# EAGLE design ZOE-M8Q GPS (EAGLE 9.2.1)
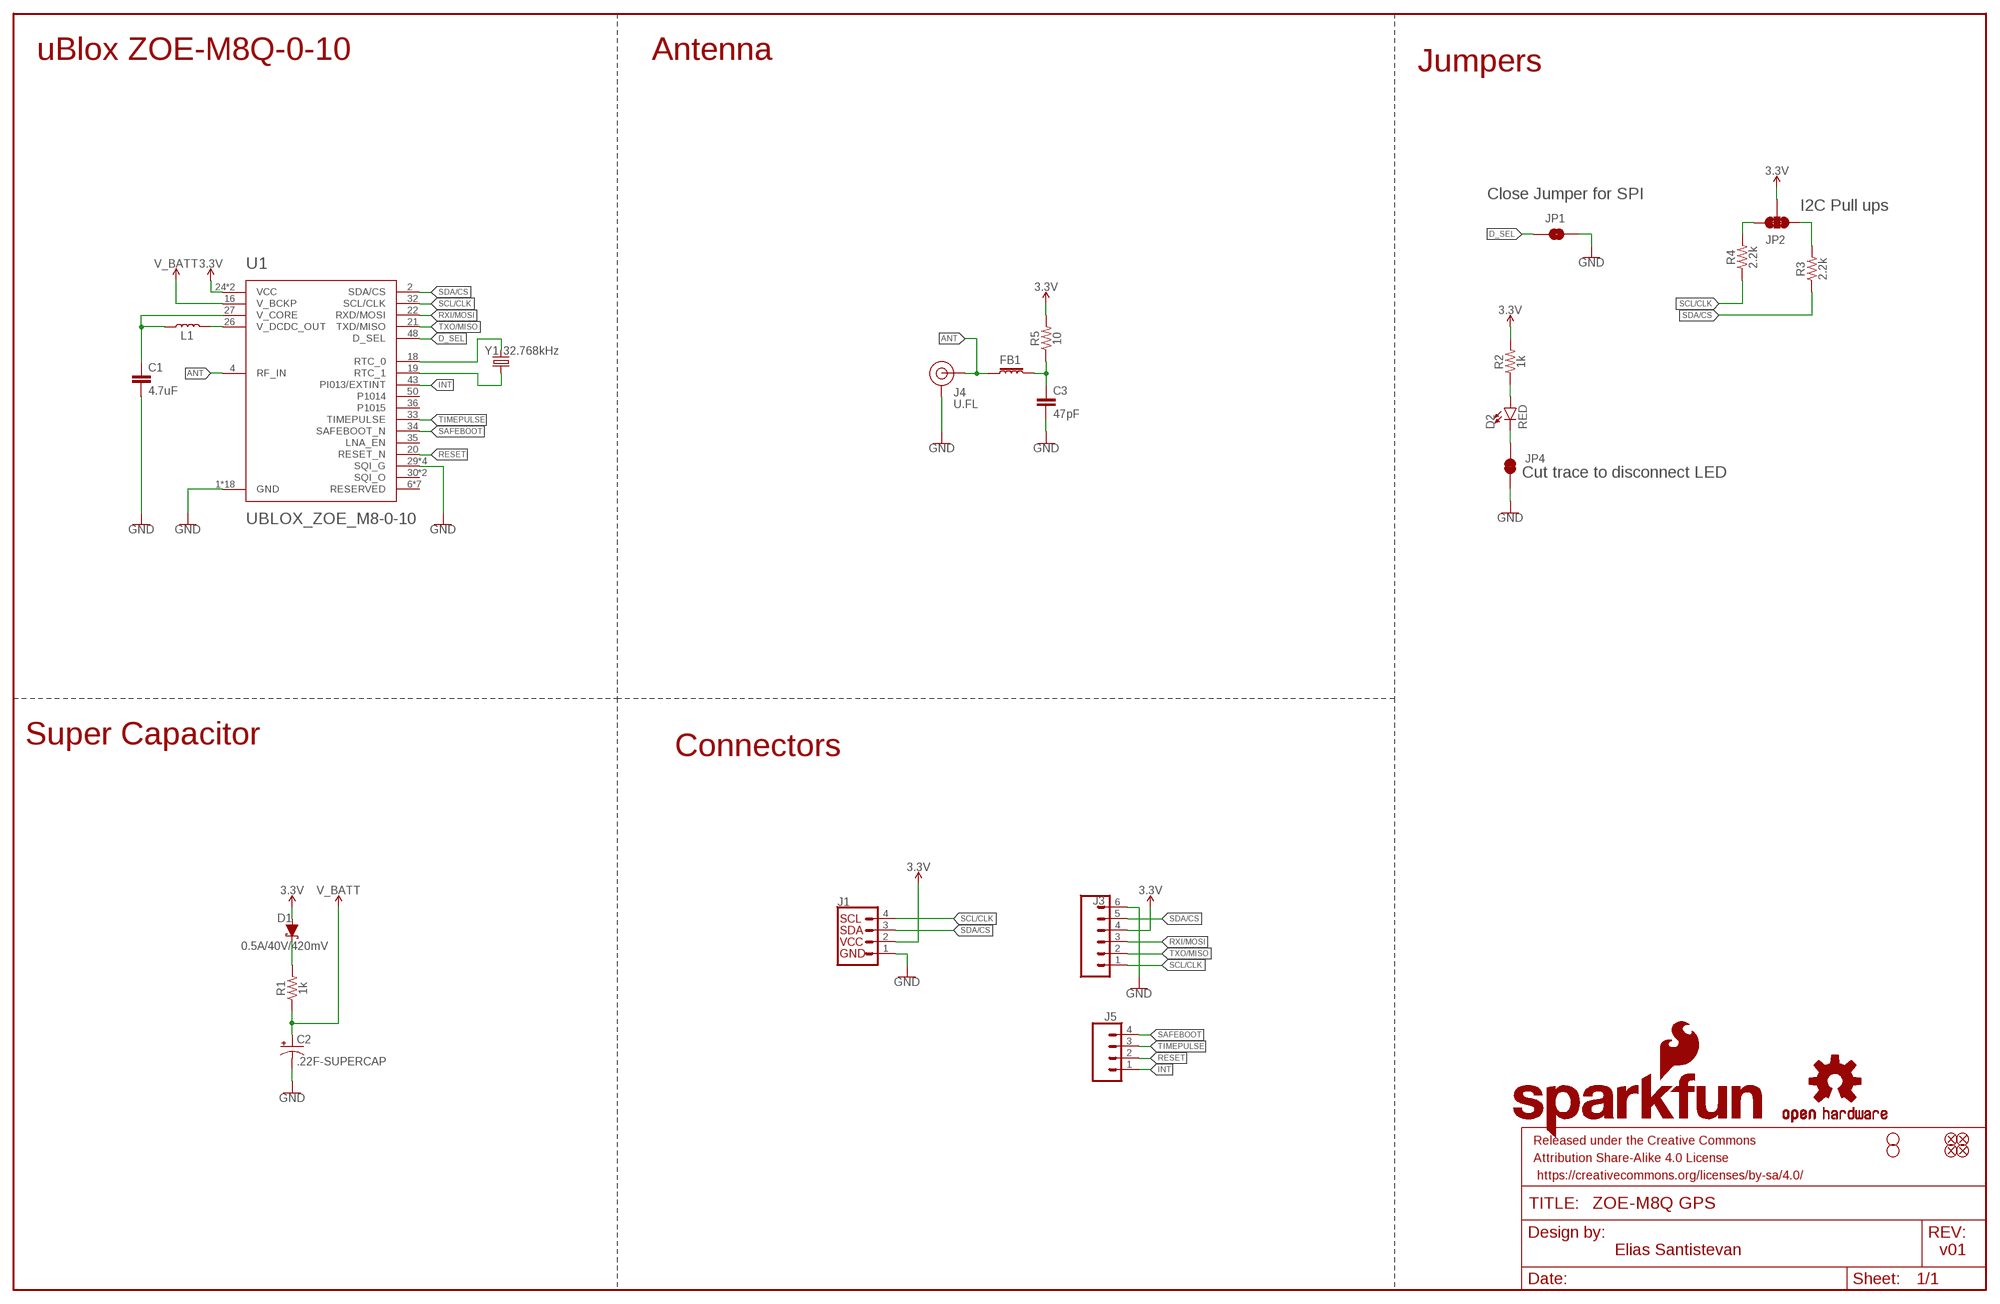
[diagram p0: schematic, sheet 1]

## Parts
C1  4.7uF  4.7UF-0603-6.3V-(10%)  [0603]
C2  .22F-SUPERCAP  [DSK-RADIAL-4.8MM]
C3  47pF  47PF-0603-50V-5%  [0603]
D1  0.5A/40V/420mV  DIODE-SCHOTTKY-PMEG4005EJ  [SOD-323]
D2  RED  LED-RED0603  [LED-0603]
FB1  FERRITE_BEAD-120_OHM-0402  [0402]
FD1  FIDUCIALUFIDUCIAL  [FIDUCIAL-MICRO]
FD2  FIDUCIALUFIDUCIAL  [FIDUCIAL-MICRO]
FD3  FIDUCIALUFIDUCIAL  [FIDUCIAL-MICRO]
FD4  FIDUCIALUFIDUCIAL  [FIDUCIAL-MICRO]
FRAME1  FRAME-LEDGER  [CREATIVE_COMMONS]
H2  STAND-OFFTIGHT  [STAND-OFF-TIGHT]
H3  STAND-OFFTIGHT  [STAND-OFF-TIGHT]
J1  QWIIC_CONNECTORJS-1MM  [JST04_1MM_RA]
J3  CONN_06NO_SILK_NO_POP  [1X06_NO_SILK]
J4  U.FL  U.FL2PIN  [U.FL]
J5  CONN_041X04_NO_SILK  [1X04_NO_SILK]
JP1  JUMPER-SMT_2_NO_SILK  [SMT-JUMPER_2_NO_SILK]
JP2  JUMPER-SMT_3_2-NC_TRACE_SILK  [SMT-JUMPER_3_2-NC_TRACE_SILK]
JP4  JUMPER-SMT_2_NC_TRACE_SILK  [SMT-JUMPER_2_NC_TRACE_SILK]
L1  2.2UH_SHIELDED_INDUCTOR  [0806_NDUC]
LOGO1  SFE_LOGO_NAME_FLAME.1_INCH  [SFE_LOGO_NAME_FLAME_.1]
LOGO2  OSHW-LOGOS  [OSHW-LOGO-S]
LOGO3  SFE_LOGO_FLAME.1_INCH  [SFE_LOGO_FLAME_.1]
R1  1k  1KOHM-0603-1/10W-1%  [0603]
R2  1k  1KOHM-0603-1/10W-1%  [0603]
R3  2.2k  2.2KOHM-0603-1/10W-1%  [0603]
R4  2.2k  2.2KOHM-0603-1/10W-1%  [0603]
R5  10  10OHM-0603-1/10W-1%  [0603]
U1  UBLOX_ZOE_M8-0-10  [UBLOX_ZOE_M8-0-10]
Y1  32.768kHz  CRYSTAL-32.768KHZSMD-3.2X1.5  [CRYSTAL-SMD-3.2X1.5MM]

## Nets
3.3V: D1.A J1.2 J3.4 JP2.2 R2.2 R5.2 U1.24(VCC) U1.25(VCC)
ANT: FB1.1 J4.FEED(SIGNAL) U1.4(RF_IN)
D_SEL: JP1.1 U1.48(D_SEL)
GND: C1.2 C2.- C3.2 J1.1 J3.6 J4.1(GND) J4.2(GND) JP1.2 JP4.1 U1.1(GND) U1.3(GND) U1.5(GND) U1.7(GND) U1.8(GND) U1.9(GND) U1.10(GND) U1.11(GND) U1.12(GND) U1.17(GND) U1.23(GND) U1.29(SQI_G) U1.31(SQI_G) U1.37(GND) U1.38(GND) U1.39(GND) U1.40(GND) U1.41(GND) U1.44(GND) U1.46(SQI_G) U1.47(SQI_G) U1.49(GND)
INT: J5.1 U1.43(PI013/EXTINT)
N$1: JP2.1 R3.2
N$2: D1.C R1.2
N$3: JP2.3 R4.2
N$4: D2.A R2.1
N$6: C1.1 L1.P$1 U1.27(V_CORE)
N$7: L1.P$2 U1.26(V_DCDC_OUT)
N$8: D2.C JP4.2
N$9: C3.1 FB1.2 R5.1
N$13: U1.18(RTC_0) Y1.P$2
N$15: U1.19(RTC_1) Y1.P$1
RESET: J5.2 U1.20(RESET_N)
RXI/MOSI: J3.3 U1.22(RXD/MOSI)
SAFEBOOT: J5.4 U1.34(SAFEBOOT_N)
SCL/CLK: J1.4 J3.1 R4.1 U1.32(SCL/CLK)
SDA/CS: J1.3 J3.5 R3.1 U1.2(SDA/CS)
TIMEPULSE: J5.3 U1.33(TIMEPULSE)
TXO/MISO: J3.2 U1.21(TXD/MISO)
V_BATT: C2.+ R1.1 U1.16(V_BCKP)
Unconnected: U1.6(RESERVED) U1.13(RESERVED) U1.14(RESERVED) U1.15(RESERVED) U1.28(RESERVED) U1.30(SQI_O) U1.35(LNA_EN) U1.36(P1015) U1.42(RESERVED) U1.45(SQI_O) U1.50(P1014) U1.51(RESERVED)

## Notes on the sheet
- uBlox ZOE-M8Q-0-10 | Antenna
- Jumpers
- Close Jumper for SPI
- I2C Pull ups
- Cut trace to disconnect LED
- Super Capacitor
- Connectors
- Elias Santistevan | v01

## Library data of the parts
C1 = SparkFun-Capacitors:4.7UF: 4.7µF ceramic capacitors; PROD_ID: CAP-08280
C2 = SparkFun-Capacitors:.22F-SUPERCAP: ELNA DSK-621 - 220mF Electric Double Layer Capacitor (EDLC/SuperCapacitor); PROD_ID: CAP-13907
C3 = SparkFun-Capacitors:47PF: 47pF ceramic capacitors; PROD_ID: CAP-08913
D1 = SparkFun-DiscreteSemi:DIODE-SCHOTTKY: Schottky diode; PROD_ID: DIO-10955
D2 = SparkFun-LED:LED-RED: Red SMD LED; PROD_ID: DIO-00819
FB1 = SparkFun-Coils:FERRITE_BEAD-120_OHM: Ferrite Bead (blocks, cores, rings, chokes, etc.); MFG_PART: BLM15HB121SN1D; PROD_ID: NDUC-14206
FD1-FD4 = SparkFun-Aesthetics:FIDUCIAL: Fiducial Alignment Points
FRAME1 = SparkFun-Aesthetics:FRAME-LEDGER: Schematic Frame - Ledger
H2 H3 = SparkFun-Hardware:STAND-OFF: Stand Off
J1 = SparkFun-Connectors:QWIIC_CONNECTOR: SparkFun I2C Standard Qwiic Connector An SMD 1mm pitch JST connector makes it easy and quick (get it? Qwiic?) to connect I2C devices to each other. The Qwiic system enables fast and solderless connection between popular platforms and various sensors and actuators. We carry 200mm, 100mm, 50mm, and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; PROD_ID: CONN-13694
J3 = SparkFun-Connectors:CONN_06: Multi connection point. Often used as Generic Header-pin footprint for 0.1 inch spaced/style header connections On any of the 0.1 inch spaced packages, you can populate with these: Break Away Headers - Straight (PRT-00116) Break Away Male Headers - Right Angle (PRT-00553) Female Headers (PRT-00115)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
J4 = SparkFun-Connectors:U.FL2PIN: SMD Antenna Connector - U.FL; PROD_ID: CONN-09193; SF_ID: WRL-09144
J5 = SparkFun-Connectors:CONN_04: Multi connection point. Often used as Generic Header-pin footprint for 0.1 inch spaced/style header connections On any of the 0.1 inch spaced packages, you can populate with these: Break Away Headers - Straight (PRT-00116) Break Away Male Headers - Right Angle (PRT-00553) Female Headers (PRT-00115)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; PROD_ID: CONN-09696
JP1 = SparkFun-Jumpers:JUMPER-SMT_2_NO: Normally open jumper
JP2 = SparkFun-Jumpers:JUMPER-SMT_3_2-NC_TRACE: Normally closed trace jumper (2 of 2 connections) This jumper has a trace between all three pads so they are normally closed (NC). Use a razor knife to open the connection(s). For best results follow the IPC guidelines for cutting traces: Cutout at least 0.063 mm (0.005 in). Remove all loose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
JP4 = SparkFun-Jumpers:JUMPER-SMT_2_NC_TRACE: Normally closed trace jumper
L1 = temp:2.2UH_SHIELDED_INDUCTOR
LOGO1 = SparkFun-Aesthetics:SFE_LOGO_NAME_FLAME: SparkFun Font Logo w/ Flame
LOGO2 = SparkFun-Aesthetics:OSHW-LOGO: Open-Source Hardware (OSHW) Logo
LOGO3 = SparkFun-Aesthetics:SFE_LOGO_FLAME: SparkFun Flame Logo
R1 R2 = SparkFun-Resistors:1KOHM: 1kΩ resistor; PROD_ID: RES-07856
R3 R4 = SparkFun-Resistors:2.2KOHM: 2.2kΩ resistor; PROD_ID: RES-08272
R5 = SparkFun-Resistors:10OHM: 10Ω resistor; PROD_ID: RES-12581
U1 = temp:UBLOX_ZOE_M8-0-10: UBLOX ZOE-M8Q-0-10 u-blox ZOE-M8 standard precision GNSS SiP (System in Package) modules feature the high performance u-blox M8 GNSS engine. ZOE-M8’s ultra-miniature form factor integrates a complete GNSS receiver including SAW filter, LNA and TCXO. Handles all GNSS systems and can simulatenously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; PROD_ID: IC-14251
Y1 = SparkFun-Clocks:CRYSTAL-32.768KHZ: 32.768kHz Crystal; PROD_ID: XTAL-13062

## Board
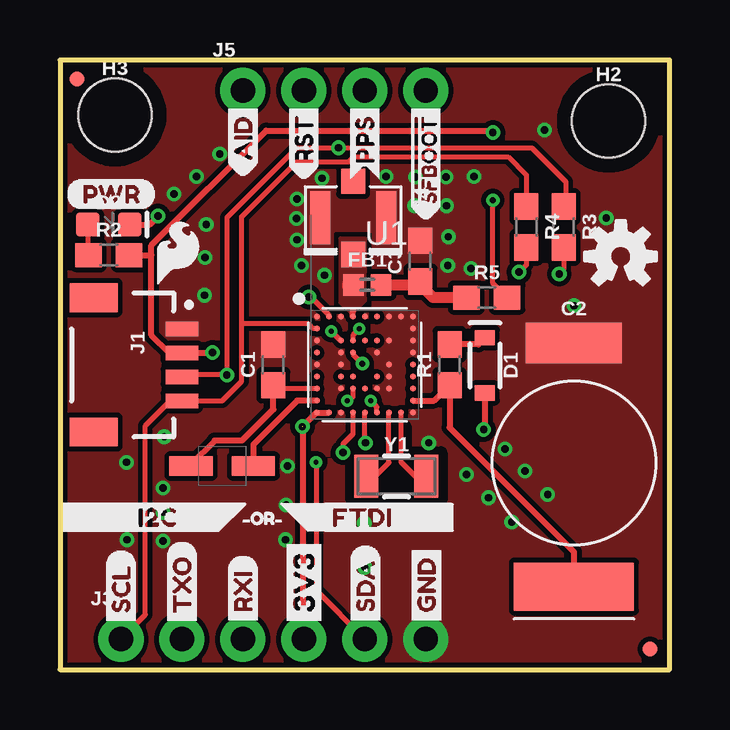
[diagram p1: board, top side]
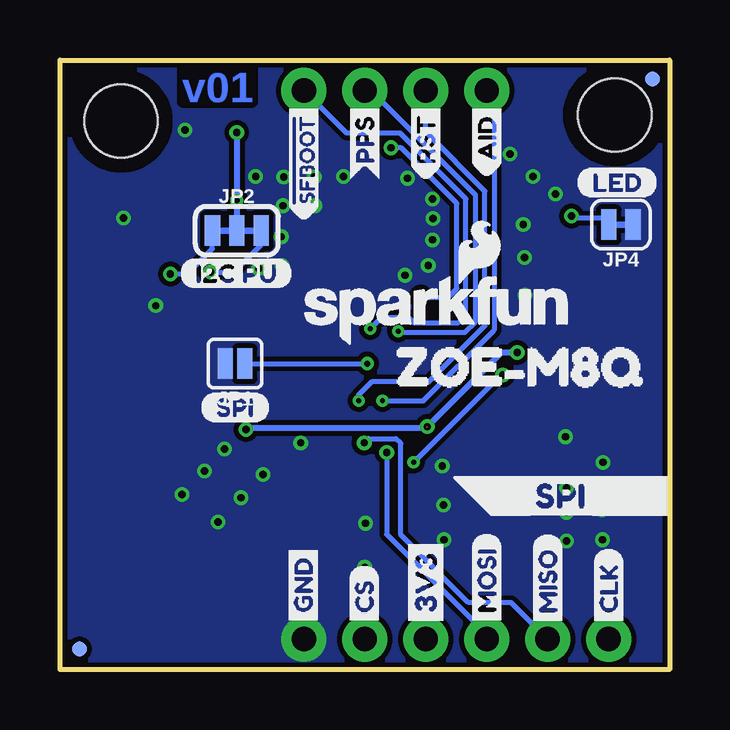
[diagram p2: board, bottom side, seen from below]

Size 25.4 x 25.4 mm. Coordinates in mm from the lower left corner, seen from the top.
Outline: 0,0 25.4,0 25.4,25.4 0,25.4 0,0
Copper layers (1*16): Top 0.035mm / dielectric 1.5mm / Bottom 0.035mm
Design rules "SparkFun-2-layer-TIGHT *": minimum track width 7mil, minimum drill 15mil, track to track 7mil, track to pad 7mil, pad to pad 7mil, via to via 7mil, smd to smd 7mil, copper to edge 7mil, drill to drill 7mil, minimum pad ring 7mil, minimum via ring 6mil, stop-mask expansion 4mil, vias tented up to drill 25mil, thermal gap 10mil
tRestrict: 7 lines

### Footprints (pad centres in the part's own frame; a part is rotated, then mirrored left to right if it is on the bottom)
0603 = smd 1.1 x 1: 1 -0.85,0; 2 0.85,0
DSK-RADIAL-4.8MM = smd 5 x 2: + 0,5.15 | smd 4 x 1.7: - 0,-5
SOD-323 = smd 0.63 x 0.83: A 1.15,0; C -1.15,0
LED-0603 = smd 1 x 1: A -0.877,0; C 0.877,0
0402 = smd 0.85 x 0.9: 1 -0.58,0; 2 0.58,0
FIDUCIAL-MICRO = smd 0.635 x 0.635: 1 0,0
STAND-OFF-TIGHT = hole 3.048: 0,0
JST04_1MM_RA = smd 0.6 x 1.35: 1 -1.5,0; 2 -0.5,0; 3 0.5,0; 4 1.5,0 | smd 1.2 x 2: NC1 2.8,-3.675; NC2 -2.8,-3.675
1X06_NO_SILK = drill 1.016 pad 1.88: 1 0,0; 2 2.54,0; 3 5.08,0; 4 7.62,0; 5 10.16,0; 6 12.7,0
U.FL = smd 2.2 x 0.85: 1 0,1.375; 2 0,-1.375 | smd 1.05 x 1: FEED 1.525,0; NC -1.525,0
1X04_NO_SILK = drill 1.016 pad 1.88: 1 0,0; 2 2.54,0; 3 5.08,0; 4 7.62,0
SMT-JUMPER_2_NO_SILK = smd 0.635 x 1.27: 1 -0.406,0; 2 0.406,0
SMT-JUMPER_3_2-NC_TRACE_SILK = smd 0.635 x 1.27: 1 -1.016,0; 2 0,0; 3 1.016,0
SMT-JUMPER_2_NC_TRACE_SILK = smd 0.635 x 1.27: 1 -0.508,0; 2 0.508,0
0806_NDUC = smd 1.8 x 0.8: P$1 -1.3,0; P$2 1.3,0
UBLOX_ZOE_M8-0-10 = smd 0.25 x 0.25: 1 -1.996,2.004; 2 -1.496,2.004; 3 -0.996,2.004; 4 -0.496,2.004; 5 0.004,2.004; 6 0.504,2.004; 7 1.004,2.004; 8 1.504,2.004; 9 2.004,2.004; 10 2.004,1.504; 11 2.004,1.004; 12 2.004,0.504; 13 2.004,0.004; 14 2.004,-0.496; 15 2.004,-0.996; 16 2.004,-1.496; 17 2.004,-1.996; 18 1.504,-1.996; 19 1.004,-1.996; 20 0.504,-1.996; 21 0.004,-1.996; 22 -0.496,-1.996; 23 -0.996,-1.996; 24 -1.496,-1.996; 25 -1.996,-1.996; 26 -1.996,-1.496; 27 -1.996,-0.996; 28 -1.996,-0.496; 29 -1.996,0.004; 30 -1.996,0.504; 31 -1.996,1.004; 32 -1.996,1.504; 33 -0.996,1.004; 34 -0.496,1.004; 35 0.004,1.004; 36 0.504,1.004; 37 1.004,1.004; 38 1.004,0.004; 39 1.004,-0.496; 40 1.004,-0.996; 41 0.504,-0.996; 42 0.004,-0.996; 43 -0.496,-0.996; 44 -0.996,-0.996; 45 -0.996,-0.496; 46 -0.996,0.004; 47 -0.996,0.504; 48 -0.496,0.504; 49 0.504,0.504; 50 0.504,-0.496; 51 -0.496,-0.496
CRYSTAL-SMD-3.2X1.5MM = smd 1 x 1.8: P$1 -1.25,0; P$2 1.25,0

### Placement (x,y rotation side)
C1  8.89,12.7 90 top
C2  21.41,8.61 180 top
C3  15.01,17.02 90 top
D1  17.7,12.67 270 top
D2  2.03,18.54 0 top
FB1  12.8,16.03 0 top
FD1  0.71,24.61 0 top
FD2  24.59,0.86 0 bottom
FD3  0.71,24.61 0 bottom
FD4  24.59,0.86 0 top
FRAME1  not placed on the board
H2  22.86,22.86 0 top
H3  2.29,23.11 0 top
J1  5.08,12.7 270 top
J3  2.54,1.27 0 top
J4  12.22,18.82 270 top
J5  7.62,24.13 0 top
JP1  18.11,12.75 180 bottom
JP2  18.03,18.29 0 bottom
JP4  2.03,18.54 180 bottom
L1  6.76,8.48 0 top
LOGO1  9.65,14.99 0 bottom
LOGO2  23.36,17.21 0 top
LOGO3  4.9,17.39 0 top
R1  16.23,12.7 90 top
R2  2.03,17.27 0 top
R3  20.98,18.44 270 top
R4  19.43,18.44 270 top
R5  17.78,15.49 0 top
U1  12.7,12.7 0 top
U$1  [3V3-03]  10.16,1.57 90 top
U$2  [SDA0]  12.73,1.7 90 top
U$3  [SCL0]  2.54,1.68 90 top
U$4  [GND0]  15.27,1.7 90 top
U$5  [CS0]  12.73,1.68 90 bottom
U$6  [MISO0]  5.08,1.65 90 bottom
U$7  [GND0]  15.27,1.7 90 bottom
U$8  [CLK0]  2.54,1.68 90 bottom
U$9  [SPI0]  6.49,7.24 0 bottom
U$10  [3V3-03]  10.16,1.57 90 bottom
U$11  [AID0]  7.62,20.52 90 bottom
U$12  [RST0]  10.16,20.37 90 bottom
U$13  [PPS0]  12.7,20.4 90 bottom
U$14  [#SFBOOT0]  15.24,18.59 90 top
U$15  [TXO0]  5.08,1.65 90 top
U$16  [ZOE#M8Q0]  12.75,12.62 0 bottom
U$17  [SPI0]  19.56,10.92 0 bottom
U$18  [I2C_PU0]  20.45,16.51 0 bottom
U$19  [RXI0]  7.62,1.7 90 top
U$21  [AID0]  7.62,20.52 90 top
U$22  [RST0]  10.16,20.37 90 top
U$23  [PPS0]  12.7,20.4 90 top
U$24  [#SFBOOT0]  15.24,18.59 90 bottom
U$25  [LED0]  3.91,20.29 0 bottom
U$26  [PWR-()-03]  0.25,19.81 0 top
U$27  [MOSI0]  7.62,1.68 90 bottom
U$28  [I2C0]  2.54,6.35 0 top
U$29  [FTDI0]  10.64,6.35 0 top
U$30  [#OR#0]  7.16,6.3 0 top
Y1  14.02,8.05 0 top

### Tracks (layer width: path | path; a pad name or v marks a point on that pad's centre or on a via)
3.3V  (via drill 0.25, 0.3)  (1 unrouted)
  Top 0.203: R5.2 18.03,16.09 v18.03,19.56
  Top 0.254: U1.24 U1.25 10.68,10.7 v10.1,10.12 | v6.35,13.21 J1.2 4.55,13.2 3.81,13.94 3.81,17.27 | D1.A 17.7,10.06 v17.65,10.01 | v18.03,22.38 17.96,22.45 8.59,22.45 3.81,17.68 3.81,17.27 | R2.2 3.81,17.27 | J3.4 10.11,1.32 v10.11,10.11
  Bottom 0.254: v6.35,13.21 7.01,13.21 v10.1,10.12 10.16,10.06 17.6,10.06 v17.65,10.01 | v18.03,22.38 v18.03,19.56 JP2.2
ANT
  Top 0.254: U1.4 12.2,14.95 12.22,14.96
  Top 0.889: 12.2,16.01 FB1.1
  pour Top (isolate 0.152, no thermals): 11.68,17.14 11.68,15.29 12.09,14.88 12.24,14.88 12.73,15.37 12.73,17.98 11.71,17.98 11.68,17.98
D_SEL  (via drill 0.25)
  Top 0.203: U1.48 12.2,13.14 v12.6,12.75
  Bottom 0.203: JP1.1 v12.6,12.75
GND  (via drill 0.3)
  other vias: 21.41,15.16 20.19,22.48 16.94,8.13 4.29,5.36 12.67,6.1 12.7,4.27 6.1,18.54 5.69,20.55 22.76,18.82 2.77,8.64 15.37,9.45 9.47,8.48 4.34,9.7 11.02,16.43 9.88,17.91 9.88,19.61 10.92,20.47 13.59,20.55 14.78,19.33 16.1,19.33 16.08,20.52 14.81,20.52 10.06,16.84 9.86,18.8 17.25,20.55 16.18,18.03 16.15,16.84 17.12,16.71 9.4,5.41 9.42,6.86 4.29,6.55 4.29,7.57 6.05,17.17 6.02,15.6 6.65,21.49 4.75,19.81 18.54,9.19 19.38,8.28 20.32,7.29 17.86,7.16 18.82,6.15 2.82,6.65 2.79,5.41
  pour Top (isolate 0.203, rank 4, no thermals): 0,25.4 0,0 25.4,0 25.4,25.4
  pour Bottom (isolate 0.203, rank 4, no thermals): 0,25.4 0,0 25.4,0 25.4,25.4
INT  (via drill 0.2)
  Top 0.203: U1.43 12.2,11.37 12.04,11.2 v11.96,11.2
  Bottom 0.203: v11.96,11.2 10.26,11.2 7.32,14.15 7.32,23.82 J5.1
N$1  (via drill 0.3)
  Top 0.203: R3.2 20.98,16.66 v20.8,16.48
  Bottom 0.203: 19.15,18.39 JP2.1 19.05,17.53 20.09,16.48 v20.8,16.48
N$2
  Top 0.254: D1.C 17.43,13.55 R1.2
N$3  (via drill 0.3)
  Top 0.203: R4.2 19.43,16.87 v19.13,16.56
  Bottom 0.203: v19.13,16.56 18.16,16.56 17.02,17.7 JP2.3
N$4
  Top 0.203: D2.A 1.16,17.3 R2.1
N$6
  Top 0.203: C1.1 9.08,11.66 9.12,11.7 U1.27
  Top 0.254: C1.1 8.89,10.85 7.58,9.54 6.44,9.54 5.46,8.55 L1.P$1
N$7
  Top 0.254: U1.26 9.88,11.2 8.06,9.38 L1.P$2
N$8  (via drill 0.3)
  Top 0.254: D2.C 3.73,18.54 v4.09,18.9
  Bottom 0.203: v4.09,18.9 3.99,18.8 2.79,18.8 JP4.2
N$9
  Top 0.457: FB1.2 15.01,16.03 | 15.01,16.03 C3.1 | R5.1 15.54,15.49 15.01,16.03
N$13
  Top 0.203: Y1.P$2 14.81,8.05 14.2,8.66 U1.18
N$15
  Top 0.203: Y1.P$1 13.13,8.05 13.7,8.62 U1.19
RESET  (via drill 0.2)
  Top 0.203: U1.20 13.2,10.95 v12.95,11.2
  Bottom 0.203: v12.95,11.2 12.95,11.46 12.42,11.99 10.03,11.99 7.7,14.33 7.7,19.94 10.16,22.4 J5.2
RXI/MOSI  (via drill 0.3)
  Top 0.203: U1.22 12.2,9.82 11.79,9.4 v11.79,9.04
  Bottom 0.203: v11.79,9.04 11.79,5.64 7.62,1.47 J3.3
SAFEBOOT  (via drill 0.2)
  Top 0.203: v12.47,14.2 12.2,13.93 U1.34
  Bottom 0.203: J5.4 13.46,22.35 11.23,22.35 8.48,19.61 8.48,14.76 8.79,14.45 10.67,14.45 10.9,14.68 11.99,14.68 v12.47,14.2
SCL/CLK
  Top 0.203: 7.57,14.35 7.57,12.01 6.75,11.2 J1.4 4.6,11.2 3.56,10.16 3.56,2.29 J3.1 | 7.57,14.35 7.57,18.87 9.86,21.16 12.04,21.16 12.24,21.36 18.67,21.36 19.43,20.6 R4.1 | U1.32 10.56,14.2 10.36,14.4 7.62,14.4 7.57,14.35
SDA/CS  (via drill 0.2, 0.3)
  Top 0.203: J1.3 5.16,12.28 v6.95,12.28 v6.96,12.28 6.96,18.85 9.86,21.74 v11.61,21.74 19.66,21.74 21.08,20.32 21.08,19.39 R3.1 | U1.2 11.2,14.78 10.46,15.52 v10.36,15.52 | v10.67,8.64 10.67,3.3 J3.5
  Bottom 0.203: 6.98,12.3 7,12.3 v10.67,8.64 | v10.36,15.52 9.22,15.52 8.87,15.88 8.87,19.43 11.18,21.74 v11.61,21.74
  Bottom 0.254: 6.98,12.3 v6.95,12.28
TIMEPULSE  (via drill 0.2)
  Top 0.203: U1.33 v11.31,14.1 v11.3,14.1
  Bottom 0.203: v11.3,14.1 11.25,14.05 8.53,14.05 8.08,14.5 8.08,19.76 12.45,24.13 J5.3
TXO/MISO  (via drill 0.3)
  Top 0.203: v12.72,9.45 12.7,9.47 U1.21
  Bottom 0.203: v12.72,9.45 12.55,9.63 11.4,9.63 11.2,9.42 11.2,5.61 8.38,2.79 6.6,2.79 J3.2
V_BATT
  Top 0.254: U1.16 15.59,11.2 R1.1 16.23,10.09 21.41,4.91 C2.+

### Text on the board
Bottom: v01
Measures: Units in Inches
tDocu: Elias Santistevan

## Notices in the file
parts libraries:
SparkFun-Aesthetics: Licensing: Creative Commons ShareAlike 4.0 International - https://creativecommons.org/licenses/by-sa/4.0
SparkFun-Aesthetics: Released under the Creative Commons Attribution Share-Alike 4.0 License
SparkFun-Aesthetics: https://creativecommons.org/licenses/by-sa/4.0
